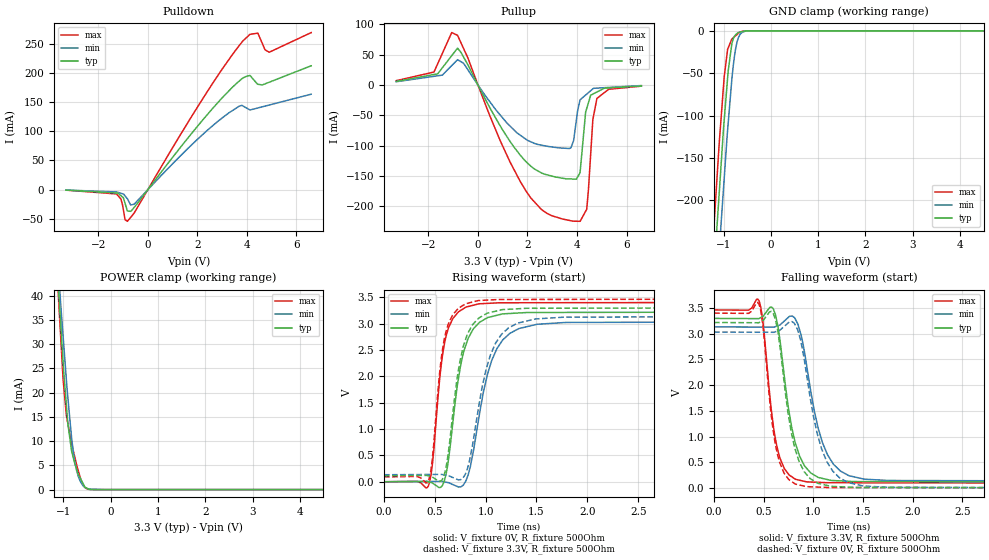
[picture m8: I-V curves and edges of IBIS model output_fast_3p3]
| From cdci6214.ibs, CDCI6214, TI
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|   output_fast_3p3 Model
[Model]   output_fast_3p3
Model_type   3-state
Polarity   Non-Inverting
Vmeas = 1.65
Vref = 0
Cref = 1pF
Rref = 100000
|   typ   min   max
C_comp   5.317E-12   5.227E-12   5.396E-12
|  Where Nom  PVT is Nominal Process, 3.3V,   32C
|   Fast PVT is Strong Process,  3.465V, -35C
|   Slow PVT is Weak Process,   3.135V,  110C
[Voltage Range]   3.3   3.135   3.465
|Junction Temperature
[Temperature Range]   32   110   -35
[Pullup Reference]   3.3   3.135   3.465
[Pulldown Reference]   -0   0   0
[Power Clamp Reference]   3.3   3.135   3.465
[GND Clamp Reference]   0   0   0
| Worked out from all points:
|   slope of the pulldown table from 0 to 0.495 V, typ, clamps not added: 17.9 ohm
|   slope of the pullup table from 0 to 0.495 V, typ, clamps not added: 12.8 ohm
|   GND clamp passes 1 mA (typ) near -0.61 V on its own axis
|   POWER clamp passes 1 mA (typ) near -0.57 V on its own axis
|   falling waveform, V_fixture 3.3V, R_fixture 500Ohm: 20-80 % time 161ps typ, 203ps min, 123ps max; typ from 3.3 V to 0.114 V
|   rising waveform, V_fixture 0V, R_fixture 500Ohm: 20-80 % time 153ps typ, 206ps min, 112ps max; typ from 0 V to 3.22 V
|   rising waveform, V_fixture 3.3V, R_fixture 500Ohm: 20-80 % time 150ps typ, 202ps min, 111ps max; typ from 0.114 V to 3.3 V
|   falling waveform, V_fixture 0V, R_fixture 500Ohm: 20-80 % time 160ps typ, 201ps min, 122ps max; typ from 3.22 V to 0 V
[Pulldown]
|   Voltage   I(typ)   I(min)   I(max)
-3.3V     -624.3uA   -515.6uA   -732.9uA
-1.265V   -5.651mA   -3.803mA   -7.198mA
-1.084V   -10.2mA    -6.051mA   -16.08mA
-987.4mV  -13.62mA   -7.309mA   -34.17mA
-823.9mV  -36.36mA   -15.42mA   -53.99mA
-559.1mV  -30.6mA    -24.83mA   -40.4mA
2.424V    129.5mA    102.4mA    169.2mA
3.836V    191.1mA    143.4mA    254.3mA
4.128V    195.5mA    136.4mA    265.7mA
4.443V    180.4mA    139.8mA    267.8mA
4.904V    183.9mA    144.9mA    235.2mA
6.6V      212mA      163.4mA    268.8mA
[GND Clamp]
|   Voltage   I(typ)   I(min)   I(max)
-3.3V     -2.319A    -2.383A    -2.268A
-1.235V   -318.2mA   -389.1mA   -258.7mA
-1.146V   -236.9mA   -310.1mA   -180.3mA
-1.054V   -160mA     -229.1mA   -104.8mA
-985.2mV  -104.7mA   -173.5mA   -53.98mA
-902.3mV  -47.57mA   -109.3mA   -20.23mA
-824.1mV  -15.03mA   -56.81mA   -9.674mA
-793.7mV  -9.33mA    -40.72mA   -8.178mA
-738.3mV  -4.241mA   -19.15mA   -5.477mA
-683.5mV  -1.95mA    -7.839mA   -2.809mA
-335.3mV  -1.438uA   -4.692uA   -408.5nA
6.6V      0A         0A         0A
[Pullup]
|   Voltage   I(typ)   I(min)   I(max)
-3.3V     5.853mA    5.289mA    7.072mA
-1.775V   17.27mA    14.27mA    21.34mA
-1.058V   48.37mA    31.98mA    86.52mA
-823.9mV  60.78mA    41.75mA    82.03mA
1.964V    -127.6mA   -90.41mA   -176.5mA
2.809V    -148.6mA   -101.4mA   -212.6mA
3.836V    -155.4mA   -95.01mA   -224.9mA
4.119V    -145.3mA   -25.41mA   -225.2mA
4.392V    -38.96mA   -15.16mA   -205.4mA
4.641V    -15.07mA   -6.442mA   -57.07mA
4.806V    -11.61mA   -5.226mA   -22.26mA
6.6V      -1.681mA   -986.2uA   -1.973mA
[POWER Clamp]
|   Voltage   I(typ)   I(min)   I(max)
-3.3V     448.6mA    388.2mA    543.9mA
-1.1V     41.23mA    44.74mA    39.27mA
-1.047V   32.97mA    37.2mA     30.18mA
-1.003V   26.09mA    31.5mA     22.64mA
-932.8mV  17.17mA    22.42mA    15.16mA
-904.2mV  13.66mA    19.09mA    13.68mA
-824.1mV  7.954mA    10.65mA    9.494mA
-757.1mV  5.417mA    5.789mA    6.729mA
-684.8mV  3.191mA    2.796mA    3.921mA
-589.2mV  1.383mA    880.3uA    1.161mA
-514mV    362.7uA    284.1uA    228.9uA
6.6V      0A         0A         0A
[Ramp]
R_load = 500
|   typ   min   max
dV/dt_r   1.93192/1.50672e-10   1.81984/2.03719e-10   2.04158/1.1209e-10
dV/dt_f   1.91169/1.58489e-10   1.80051/2.00555e-10   2.02331/1.22363e-10
[Falling Waveform]
V_fixture = 3.3V
V_fixture_min = 3.135V
V_fixture_max = 3.465V
R_fixture = 500Ohm
C_fixture = 0F
|   Time   V(typ)   V(min)   V(max)
0s        3.3V       3.134V     3.465V
451.4ps   3.296V     3.131V     3.648V
489.4ps   3.336V     3.131V     3.272V
617.6ps   3.373V     3.139V     952.9mV
705.4ps   2.196V     3.246V     381.7mV
819.4ps   859.7mV    3.281V     167.5mV
911.6ps   425mV      2.625V     125.7mV
1.09ns    184mV      885.3mV    104.1mV
1.357ns   127.4mV    237.4mV    99.82mV
4ns       113.7mV    133.4mV    92.78mV
[Rising Waveform]
V_fixture = 0V
V_fixture_min = 0V
V_fixture_max = 0V
R_fixture = 500Ohm
C_fixture = 0F
|   Time   V(typ)   V(min)   V(max)
0s        122.1uV    494.8uV    17.64uV
436.4ps   55.4uV     5.278mV    -81.02mV
476.4ps   -23.98mV   5.717mV    328.5mV
574.6ps   -71.82mV   4.111mV    2.384V
624.6ps   286.8mV    -12.93mV   2.857V
677.4ps   1.121V     -52.8mV    3.096V
805.4ps   2.593V     15.26mV    3.313V
1.058ns   3.134V     2.292V     3.388V
1.326ns   3.202V     2.906V     3.396V
4ns       3.22V      3.034V     3.403V
[Rising Waveform]
V_fixture = 3.3V
V_fixture_min = 3.135V
V_fixture_max = 3.465V
R_fixture = 500Ohm
C_fixture = 0F
|   Time   V(typ)   V(min)   V(max)
0s        113.7mV    133.4mV    92.78mV
435.4ps   114mV      138.1mV    9.557mV
474.4ps   92.03mV    138.5mV    404.8mV
573.6ps   42.95mV    136.9mV    2.479V
620.6ps   381.7mV    121.2mV    2.919V
674.4ps   1.247V     82.8mV     3.162V
802.4ps   2.696V     154.2mV    3.376V
1.046ns   3.212V     2.399V     3.45V
1.313ns   3.282V     3.009V     3.459V
4ns       3.3V       3.134V     3.465V
[Falling Waveform]
|Gnd
V_fixture = 0V
V_fixture_min = 0V
V_fixture_max = 0V
R_fixture = 500Ohm
C_fixture = 0F
|   Time   V(typ)   V(min)   V(max)
0s        3.22V      3.034V     3.403V
451.4ps   3.217V     3.03V      3.58V
488.4ps   3.254V     3.03V      3.209V
569.4ps   3.432V     3.03V      1.516V
616.6ps   3.286V     3.038V     856.8mV
702.4ps   2.101V     3.138V     294mV
816.4ps   747.6mV    3.174V     75.83mV
1.082ns   72.43mV    760mV      11.91mV
1.348ns   14.21mV    104.9mV    6.809mV
4ns       121.5uV    494.6uV    17.31uV
